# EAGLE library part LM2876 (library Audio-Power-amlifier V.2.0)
LM2876 Overture™ Audio Power Amplifier Series High-Performance 40W Audio Power Amplifier w/Mute
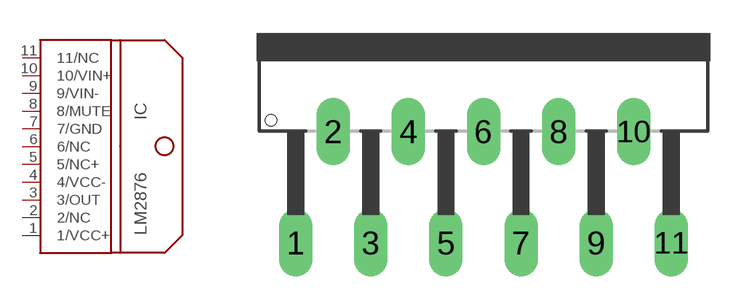
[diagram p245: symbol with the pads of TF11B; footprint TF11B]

Designator prefix IC

## LM2876  [TF11B]
1  1/VCC+  pwr
2  2/NC  nc
3  3/OUT  out
4  4/VCC-  pwr
5  5/NC+  nc
6  6/NC  nc
7  7/GND  pwr
8  8/MUTE  in
9  9/VIN-  in
10  10/VIN+  in
11  11/NC  nc

## Footprint TF11B (pad centres in mm)
TO-220 11 lead, National Semiconductor
drill 1.016 long: 1 -8.509,-9.525; 2 -6.807,-4.47; 3 -5.105,-9.525; 4 -3.404,-4.47; 5 -1.702,-9.525; 6 0,-4.47; 7 1.702,-9.525; 8 3.404,-4.47; 9 5.105,-9.525; 10 6.807,-4.47; 11 8.509,-9.525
